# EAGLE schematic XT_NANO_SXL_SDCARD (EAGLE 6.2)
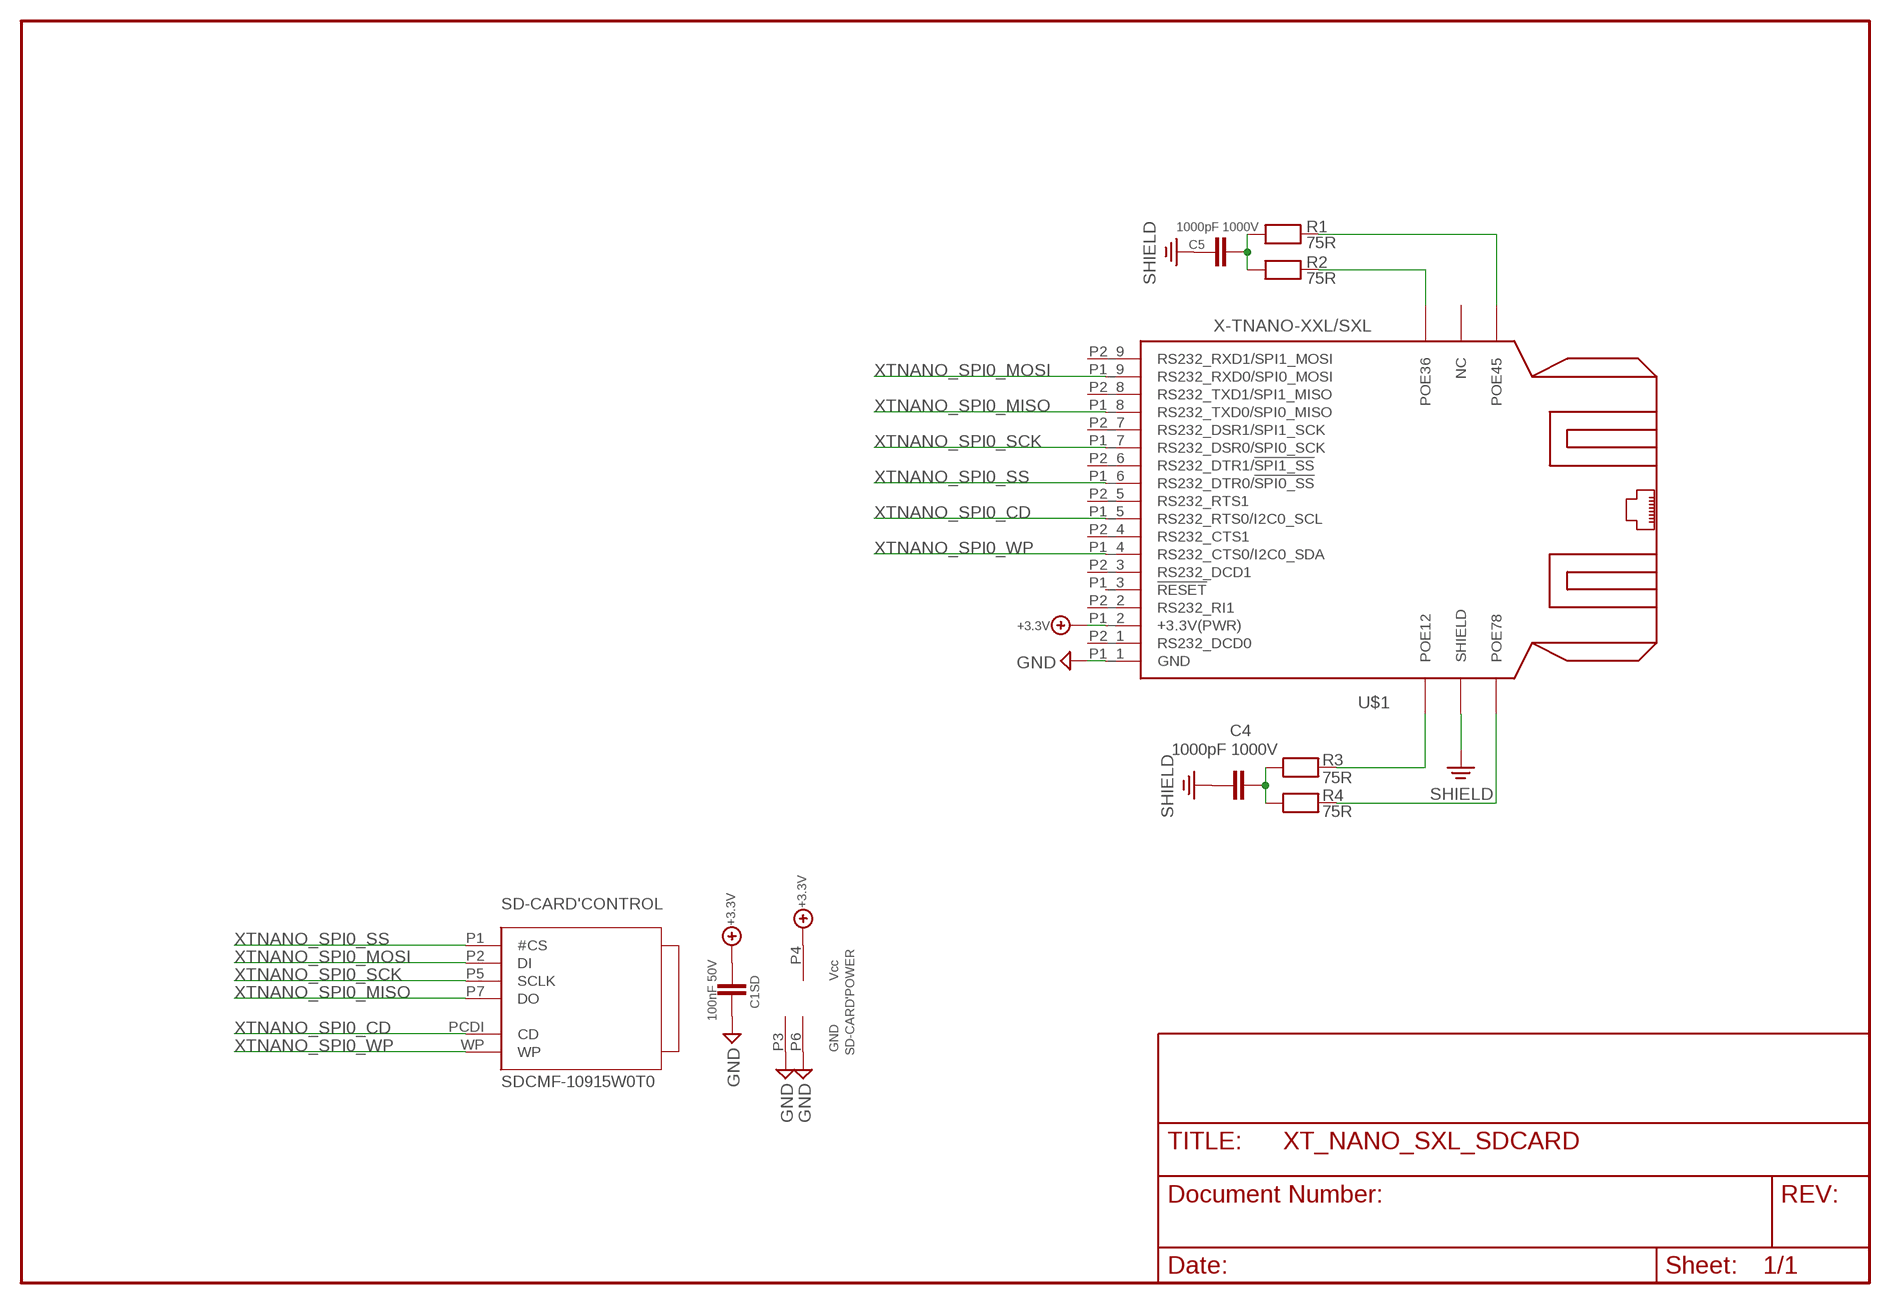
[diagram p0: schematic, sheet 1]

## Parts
C1SD  100nF 50V  CHIP-C-0603  [SMD-0603]
C4  1000pF 1000V  CHIP-C-1210  [SMD-1210]
C5  1000pF 1000V  CHIP-C-1210  [SMD-1210]
R1  75R  CHIP-R-0603  [SMD-0603]
R2  75R  CHIP-R-0603  [SMD-0603]
R3  75R  CHIP-R-0603  [SMD-0603]
R4  75R  CHIP-R-0603  [SMD-0603]
SD-CARD  SDCMF-10915W0T0  SDCMF-109XXW010SDCMF-10915W0T1_SO  [SDCMF-10915W0T1]
U$1  X-TNANO-XXL/SXL  [XT-NANO-XXL/SXL]

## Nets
+3.3V: C1SD.2 SD-CARD.P4('POWER:VCC) U$1.P1_2(+3.3V(PWR))
GND: C1SD.1 SD-CARD.P3('POWER:GND) SD-CARD.P6('POWER:GND) U$1.P1_1(GND)
N$1: C5.1 R1.1 R2.1
N$2: C4.2 R3.1 R4.1
N$4: R2.2 U$1.POE36
N$6: R1.2 U$1.POE45
N$20: R3.2 U$1.POE12
N$21: R4.2 U$1.POE78
SHIELD: C4.1 C5.2 U$1.SHIELD
XTNANO_SPI0_CD: SD-CARD.PCDI('CONTROL:CD) U$1.P1_5(RS232_RTS0/I2C0_SCL)
XTNANO_SPI0_MISO: SD-CARD.P7('CONTROL:DO) U$1.P1_8(RS232_TXD0/SPI0_MISO)
XTNANO_SPI0_MOSI: SD-CARD.P2('CONTROL:DI) U$1.P1_9(RS232_RXD0/SPI0_MOSI)
XTNANO_SPI0_SCK: SD-CARD.P5('CONTROL:SCLK) U$1.P1_7(RS232_DSR0/SPI0_SCK)
XTNANO_SPI0_SS: SD-CARD.P1('CONTROL:#CS) U$1.P1_6(RS232_DTR0/!SPI0_SS!)
XTNANO_SPI0_WP: SD-CARD.WP('CONTROL:WP) U$1.P1_4(RS232_CTS0/I2C0_SDA)
Unconnected: U$1.FLASH(NC) U$1.P1_3(!RESET) U$1.P2_1(RS232_DCD0) U$1.P2_2(RS232_RI1) U$1.P2_3(RS232_DCD1) U$1.P2_4(RS232_CTS1) U$1.P2_5(RS232_RTS1) U$1.P2_6(RS232_DTR1/!SPI1_SS!) U$1.P2_7(RS232_DSR1/SPI1_SCK) U$1.P2_8(RS232_TXD1/SPI1_MISO) U$1.P2_9(RS232_RXD1/SPI1_MOSI)

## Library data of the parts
C1SD = mea-lib:CHIP-C-?: Chip capacitance
C4 C5 = XTMACRO:CHIP-C-?: Chip capacitance
R1-R4 = XTMACRO:CHIP-R-?: Chip resistors
SD-CARD = sdcards:SDCMF-109XXW010: KingFont SD-CARD SDCMF-109XXW010 SPI -MODE
U$1 = ak-devices:X-TNANO-XXL/SXL: AK-NORD XT-NANO-XXL/SXL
